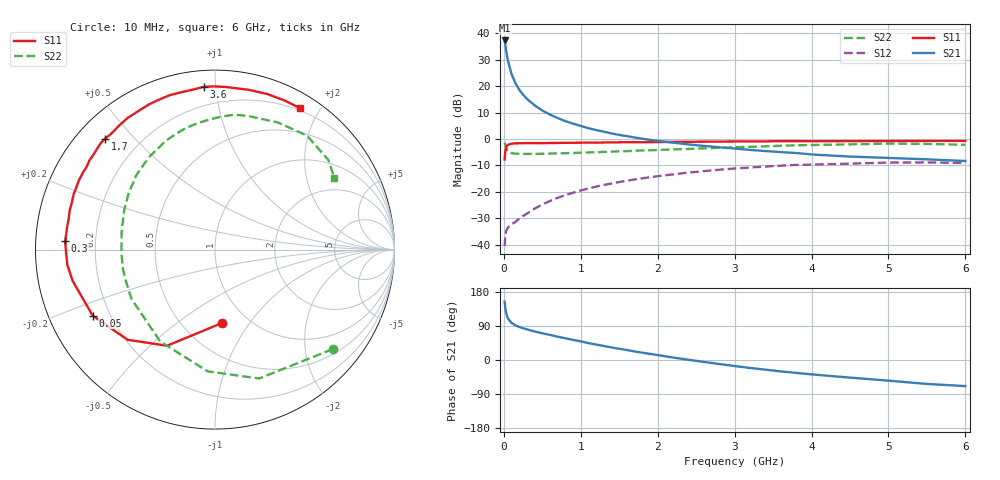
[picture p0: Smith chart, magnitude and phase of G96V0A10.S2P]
! SIEMENS Small Signal Semiconductors
! BFG235
! Si NPN RF Bipolar Junction Transistor in SOT223
! VCE = 6 V  IC = 100 mA
! Common Emitter S-Parameters:  July  1994
# GHz  S  MA  R  50
!  f  S11  S21  S12  S22
! GHz  MAG  ANG  MAG  ANG  MAG  ANG  MAG  ANG
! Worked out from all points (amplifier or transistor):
!   40 points, 10 MHz to 6 GHz, reference 50 ohm
!   highest |S21| = 37.3 dB at 10 MHz (marker M1)
!   |S21| within 3 dB of that: start of sweep to 25.68 MHz
!   unconditionally stable (mu >= 1): 459.6 MHz to 1.429 GHz
!   at 200 MHz: K = 0.77, MSG = 24.4 dB, |S12| = -30.2 dB
!   at 1.5 GHz: K = 0.99, MSG = 8.9 dB, |S12| = -16.3 dB
!   at 6 GHz: K = 0.90, MSG = 0.4 dB, |S12| = -9.1 dB
!   S11 on the Smith chart (normalised r, x): 10 MHz: 0.77, -0.75; 50 MHz: 0.14, -0.25; 300 MHz: 0.09, +0.03; 1.7 GHz: 0.08, +0.41; 3.6 GHz: 0.09, +0.93; 6 GHz: 0.17, +1.76
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0.01  0.4103 -84.3  73.55 154.3  0.0093 65.6  0.8587 -40.2
0.02  0.5985 -116.5  59.23 135.8  0.0152 50.7  0.7591 -71.1
0.03  0.6996 -134.1  47.21 123.9  0.018 42.7  0.6796 -93.4
0.05  0.7742 -151.6  31.9 110.7  0.0208 35.3  0.5961 -120.8
0.1  0.8118 -167.5  16.98 97.8  0.0241 34.8  0.5403 -149.5
0.15  0.8271 -174.1  11.43 91.4  0.0267 40.8  0.5263 -161.6
0.2  0.8286 -177.8  8.563 87.3  0.0308 45.1  0.5237 -168.4
0.25  0.8326 178.9  6.897 83.7  0.0346 48.3  0.5208 -173.0
0.3  0.8355 176.6  5.761 80.9  0.0386 51.5  0.5213 -176.8
0.4  0.8336 171.8  4.338 75.3  0.0478 54.5  0.5214 178.0
0.5  0.8334 168.1  3.459 70.5  0.0572 56.4  0.5245 173.6
0.6  0.8384 164.9  2.89 66.3  0.0669 56.6  0.5287 169.8
0.8  0.8459 158.6  2.176 57.3  0.0865 55.7  0.5365 163.1
1.1  0.8519 149.5  1.599 44.5  0.1153 51.4  0.5557 154.2
1.4  0.859 142.1  1.273 33.2  0.1433 46.0  0.5761 146.1
1.7  0.8708 134.8  1.068 22.5  0.1711 39.9  0.5989 138.2
2.2  0.8801 123.6  0.85 6.5  0.2136 29.0  0.6344 124.7
3.2  0.8967 102.1  0.62 -21.0  0.288 5.8  0.7094 98.4
3.6  0.9094 93.8  0.564 -30.1  0.3113 -4.2  0.7421 87.1
4.5  0.9101 78.0  0.464 -46.5  0.3414 -24.3  0.79 63.8
5.5  0.917 64.7  0.411 -63.2  0.3599 -46.4  0.805 38.2
6  0.9192 58.8  0.382 -68.8  0.35 -54.7  0.7748 30.8
